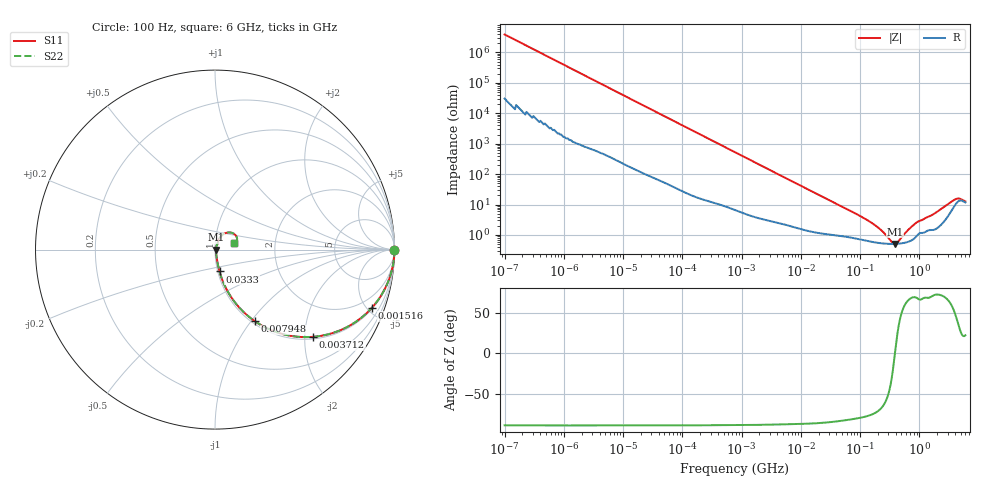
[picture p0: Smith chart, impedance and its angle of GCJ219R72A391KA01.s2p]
!Murata Part Number: GCJ219R72A391KA01
!These Parameters are Measured in Series Mode Connection
!Data Generated on Mar 13, 2026
!  o--ll--o
!Port1  Port2
!  o------o
!Operation Temp=25[degC], DC Bias Voltage=0[V]
!Freq. Start=100[Hz] Stop=6[GHz] 401[Steps]
# Hz S RI R 50
!Freq.(Hz) S11(Real) S11(Imag) S21(Real) S21(Imag) S12(Real) S12(Imag) S22(Real) S22(Imag)
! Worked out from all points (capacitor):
!   401 points, 100 Hz to 6 GHz, reference 50 ohm
!   read as one part in series: C = 406 pF near 109 Hz
!   lowest |Z| = 510 mohm at 390.8 MHz (marker M1)
!   series resonance near 388.1 MHz, so ESL is about 410 pH
!   S11 on the Smith chart (normalised r, x): 100 Hz: open; 1.516 MHz: 1.08, -5.36; 3.712 MHz: 1.05, -2.21; 7.948 MHz: 1.04, -1.04; 33.3 MHz: 1.02, -0.25; 6 GHz: 1.23, +0.10
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100  1 -2.56e-05  2e-07 2.56e-05  2e-07 2.56e-05  1 -2.56e-05
401  1 -0.000102  6e-07 0.000102  6e-07 0.000102  1 -0.000102
2008  1 -0.000509  2.5e-06 0.000509  2.5e-06 0.000509  1 -0.000509
40335  0.9998 -0.0101  0.000167 0.0101  0.000167 0.0101  0.9998 -0.0101
241822  0.9959 -0.0599  0.00411 0.0599  0.00411 0.0599  0.9959 -0.0599
774597  0.9625 -0.1838  0.0375 0.1838  0.0375 0.1838  0.9625 -0.1838
1516199  0.8741 -0.3242  0.1259 0.3242  0.1259 0.3242  0.8741 -0.3242
3712478  0.5477 -0.4859  0.4523 0.4859  0.4523 0.4859  0.5477 -0.4859
7947587  0.2212 -0.3984  0.7788 0.3984  0.7788 0.3984  0.2212 -0.3984
1.555665e7  0.0772 -0.2444  0.9228 0.2444  0.9228 0.2444  0.0772 -0.2444
3.330331e7  0.0252 -0.1218  0.9748 0.1218  0.9748 0.1218  0.0252 -0.1218
1.526266e8  0.00661 -0.0249  0.9934 0.0249  0.9934 0.0249  0.00661 -0.0249
2.283698e8  0.00547 -0.0131  0.9945 0.0131  0.9945 0.0131  0.00547 -0.0131
3.124326e8  0.0051 -0.00522  0.9949 0.00522  0.9949 0.00522  0.0051 -0.00522
3.908258e8  0.00507 0.000175  0.9949 -0.000175  0.9949 -0.000175  0.00507 0.000175
4.274388e8  0.00513 0.00234  0.9949 -0.00234  0.9949 -0.00234  0.00513 0.00234
6.395615e8  0.00603 0.0128  0.994 -0.0128  0.994 -0.0128  0.00603 0.0128
9.150511e8  0.00995 0.0241  0.9901 -0.0241  0.9901 -0.0241  0.00995 0.0241
1.712697e9  0.0163 0.0439  0.9837 -0.0439  0.9837 -0.0439  0.0163 0.0439
3.8344e9  0.087 0.0951  0.913 -0.0951  0.913 -0.0951  0.087 0.0951
4.586474e9  0.1202 0.0717  0.8798 -0.0717  0.8798 -0.0717  0.1202 0.0717
6e9  0.1067 0.039  0.8933 -0.039  0.8933 -0.039  0.1067 0.039
